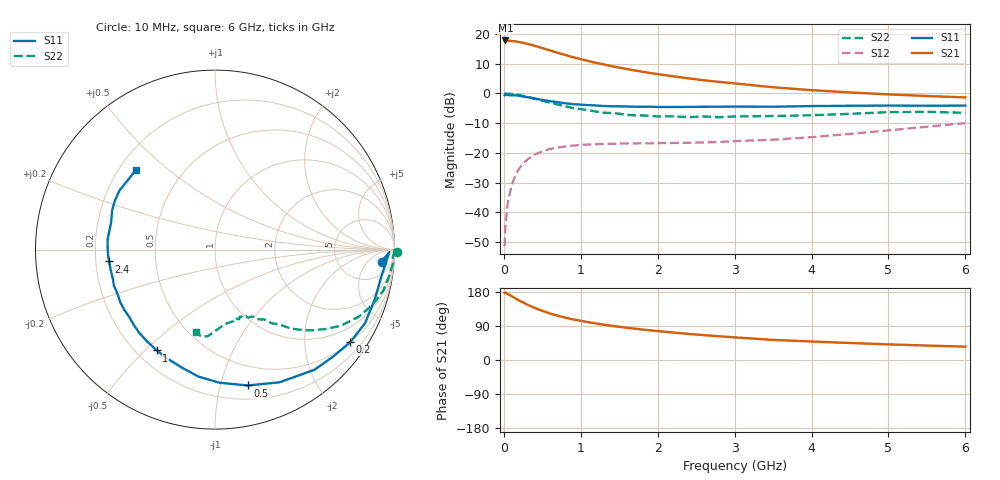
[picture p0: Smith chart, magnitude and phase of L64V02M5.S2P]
!  INFINEON TECHNOLOGIES Small Signal Semiconductors
! BFR380L3 , Si-NPN RF-Transistor in TSLP-3-1
!  Vce=4 V,  Ic=2.5 mA
! Common Emitter S-Parameters:  07. March 2005
#  GHz  S  MA  R  50
! f  S11  S21  S12  S22
! GHz  Mag  Ang  Mag  Ang  Mag  Ang  Mag  Ang
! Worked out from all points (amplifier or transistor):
!   36 points, 10 MHz to 6 GHz, reference 50 ohm
!   highest |S21| = 17.8 dB at 20 MHz (marker M1)
!   |S21| within 3 dB of that: start of sweep to 554.8 MHz
!   unconditionally stable (mu >= 1): 2.76 GHz to 4.61 GHz
!   at 250 MHz: K = 0.10, MSG = 20.3 dB, |S12| = -23.6 dB
!   at 1.4 GHz: K = 0.58, MSG = 13.0 dB, |S12| = -16.9 dB
!   at 6 GHz: K = 0.89, MSG = 4.3 dB, |S12| = -10.0 dB
!   S11 on the Smith chart (normalised r, x): 10 MHz: 14, -14; 200 MHz: 0.51, -3.15; 500 MHz: 0.32, -1.22; 1 GHz: 0.28, -0.54; 2.4 GHz: 0.26, -0.05; 6 GHz: 0.27, +0.39
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0.01  0.9309 -4.1  7.751 177.2  0.0027 81.6  1.015 -0.9
0.02  0.9719 -0.8  7.786 178.1  0.0057 93.9  0.9917 -1.9
0.05  0.9393 -8.9  7.722 174.2  0.0144 86.9  0.9937 -4.6
0.1  0.9325 -17.1  7.622 168.6  0.0284 81.2  0.9799 -9.1
0.15  0.9312 -26.2  7.526 162.8  0.0424 75.7  0.965 -13.6
0.2  0.9127 -34.5  7.326 157.0  0.0547 71.7  0.9421 -17.4
0.3  0.8691 -50.4  6.854 146.6  0.0763 63.4  0.8832 -25.1
0.4  0.822 -64.1  6.343 137.5  0.0937 56.3  0.8169 -31.4
0.5  0.7785 -76.5  5.799 129.8  0.1063 51.0  0.7552 -35.9
0.6  0.742 -88.1  5.286 122.6  0.1166 46.4  0.6999 -40.0
0.7  0.714 -97.3  4.825 117.0  0.1234 43.2  0.6512 -43.3
0.8  0.6828 -105.7  4.436 111.7  0.1282 40.3  0.6071 -46.3
1  0.6486 -120.0  3.77 103.5  0.1357 36.6  0.5451 -49.6
1.1  0.6361 -126.5  3.505 99.6  0.1385 35.2  0.5218 -52.1
1.3  0.6161 -137.7  3.078 93.3  0.1424 33.7  0.4742 -54.9
1.6  0.6037 -151.0  2.572 85.0  0.1444 32.8  0.4369 -59.7
2.2  0.592 -168.7  1.945 72.4  0.1471 35.7  0.4128 -66.2
2.4  0.5936 -173.6  1.793 68.9  0.1481 37.7  0.3983 -69.6
3.5  0.5984 165.2  1.271 53.1  0.1667 49.5  0.417 -81.2
4.5  0.6204 154.2  1.04 44.9  0.2089 60.3  0.4542 -90.0
5.5  0.621 142.1  0.905 38.1  0.2756 64.8  0.4906 -98.8
6  0.6252 135.1  0.859 35.2  0.3173 64.7  0.4729 -103.2
